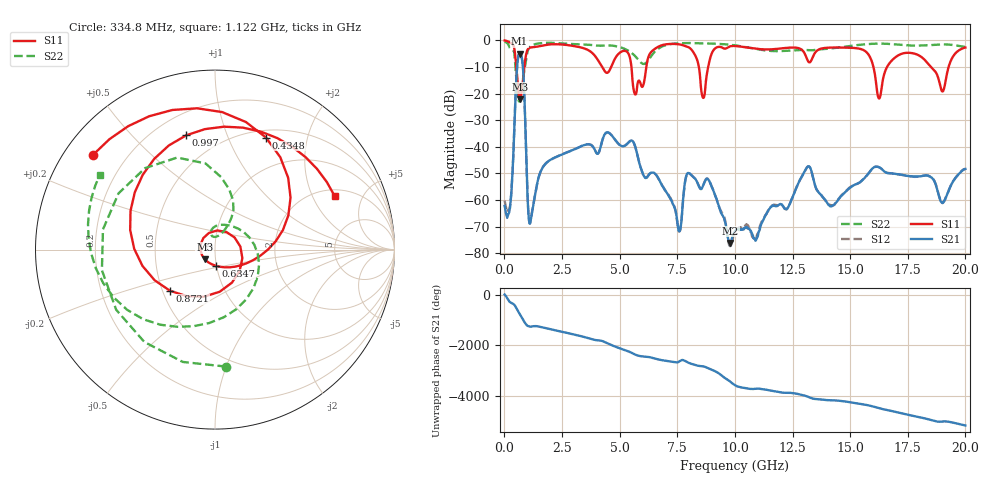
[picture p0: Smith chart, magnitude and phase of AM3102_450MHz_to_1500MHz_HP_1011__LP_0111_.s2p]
!Agilent Technologies,E8364B,MY43040894,A.07.50.67
!Agilent E8364B: A.07.50.67
!Date: Thursday, January 11, 2018 06:24:42
!Correction: S11(Full 2 Port(1,2))
!S21(Full 2 Port(1,2))
!S12(Full 2 Port(1,2))
!S22(Full 2 Port(1,2))
!S2P File: Measurements: S11, S21, S12, S22:
# Hz S  dB  R 50
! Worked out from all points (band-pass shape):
!   1601 points, 10 MHz to 20 GHz, reference 50 ohm
!   highest |S21| = -4.97 dB at 659.7 MHz (marker M1); lowest = -76.1 dB at 9.805 GHz (marker M2)
!   |S21| within 3 dB of the highest: 573.8 MHz to 781.1 MHz (207.3 MHz wide, 30.6 % of centre)
!   lowest |S11| = -22.1 dB at 672.2 MHz (marker M3), VSWR 1.17, Z = 44.3 - j4.76 ohm
!   |S11| at or under -10 dB: 5.512 GHz to 6.158 GHz (646.1 MHz wide, 11.1 % of centre); 16.01 GHz to 16.6 GHz (592 MHz wide, 3.63 % of centre); 18.51 GHz to 19.27 GHz (765.1 MHz wide, 4.05 % of centre)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
!   |S22| runs from -23.0 to -0.4 dB; largest |S21 - S12| = 0.0014
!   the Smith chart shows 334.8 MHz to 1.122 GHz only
!   S11 on the Smith chart (normalised r, x): 334.8 MHz: 0.08, +0.34; 434.8 MHz: 0.59, +1.38; 634.7 MHz: 0.99, -0.18; 872.1 MHz: 0.55, -0.28; 997 MHz: 0.32, +0.73; 1.122 GHz: 2.33, +2.98
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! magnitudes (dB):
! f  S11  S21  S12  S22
! 10 MHz  0.0  -62.2  -60.2  -0.4
! 334.8 MHz  -1.3  -52.5  -52.7  -3.7
! 434.8 MHz  -3.3  -31.9  -32.0  -5.1
! 634.7 MHz  -20.9  -5.1  -5.2  -23.0
! 659.7 MHz  -21.9  -5.0  -5.0  -22.4
! 672.2 MHz  -22.1  -5.0  -5.0  -21.6
! 872.1 MHz  -9.4  -22.0  -22.0  -11.0
! 997 MHz  -3.7  -56.8  -56.7  -4.5
! 1.122 GHz  -2.7  -68.6  -68.3  -2.3
! 3.346 GHz  -2.7  -39.7  -39.7  -1.5
! 5.67 GHz  -20.3  -39.8  -39.7  -5.9
! 6.682 GHz  -2.4  -51.8  -51.8  -3.1
! 7.581 GHz  -1.5  -71.7  -71.8  -1.1
! 7.944 GHz  -2.4  -49.9  -49.9  -1.0
! 8.618 GHz  -21.6  -54.6  -54.6  -1.1
! 9.805 GHz  -2.2  -76.1  -77.2  -1.7
! 10.01 GHz  -2.1  -71.8  -71.9  -1.9
! 13.34 GHz  -7.1  -49.8  -49.8  -3.7
! 14.18 GHz  -2.7  -62.4  -62.0  -3.0
! 16.68 GHz  -9.0  -49.9  -49.9  -1.3
! 19.01 GHz  -19.2  -61.1  -61.1  -1.5
! 20 GHz  -2.7  -48.3  -48.2  -2.5
